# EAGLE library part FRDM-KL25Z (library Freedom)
For creating FRDM-KL25Z shields
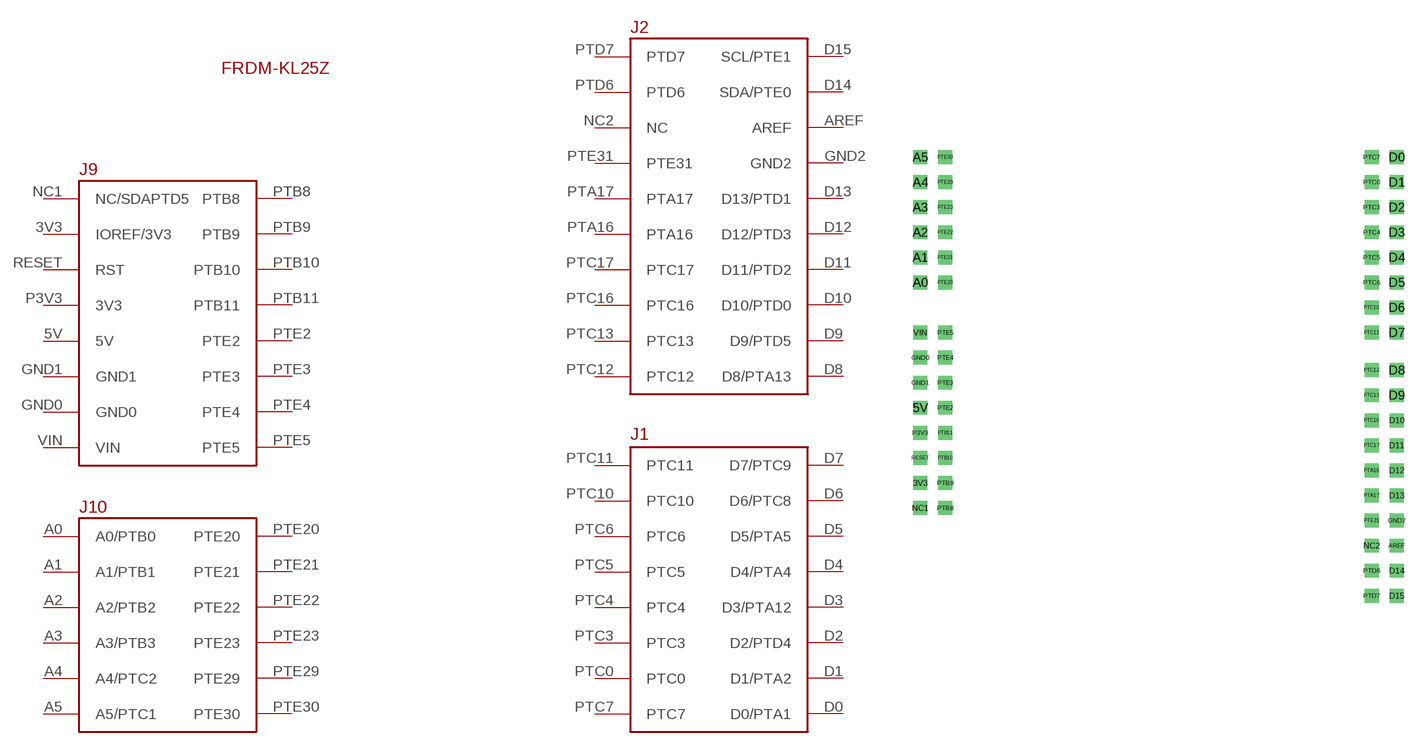
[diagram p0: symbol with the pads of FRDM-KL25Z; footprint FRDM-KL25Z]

Designator prefix FRDM

## FRDM-KL25ZARDUINO  [FRDM-KL25Z]
3V3  IOREF/3V3
5V  5V
A0  A0/PTB0
A1  A1/PTB1
A2  A2/PTB2
A3  A3/PTB3
A4  A4/PTC2
A5  A5/PTC1
AREF  AREF
D0  D0/PTA1
D1  D1/PTA2
D2  D2/PTD4
D3  D3/PTA12
D4  D4/PTA4
D5  D5/PTA5
D6  D6/PTC8
D7  D7/PTC9
D8  D8/PTA13
D9  D9/PTD5
D10  D10/PTD0
D11  D11/PTD2
D12  D12/PTD3
D13  D13/PTD1
D14  SDA/PTE0
D15  SCL/PTE1
GND0  GND0
GND1  GND1
GND2  GND2
NC1  NC/SDAPTD5
NC2  NC
P3V3  3V3
PTA16  PTA16
PTA17  PTA17
PTB8  PTB8
PTB9  PTB9
PTB10  PTB10
PTB11  PTB11
PTC0  PTC0
PTC3  PTC3
PTC4  PTC4
PTC5  PTC5
PTC6  PTC6
PTC7  PTC7
PTC10  PTC10
PTC11  PTC11
PTC12  PTC12
PTC13  PTC13
PTC16  PTC16
PTC17  PTC17
PTD6  PTD6
PTD7  PTD7
PTE2  PTE2
PTE3  PTE3
PTE4  PTE4
PTE5  PTE5
PTE20  PTE20
PTE21  PTE21
PTE22  PTE22
PTE23  PTE23
PTE29  PTE29
PTE30  PTE30
PTE31  PTE31
RESET  RST
VIN  VIN

## Footprint FRDM-KL25Z (pad centres in mm)
Use straight headers (2 6-pin and 2 8-pin) to connect to an Arduino
drill 0.9 square: 3V3 -22.86,-8.89; 5V -22.86,-1.27; A0 -22.86,11.43; A1 -22.86,13.97; A2 -22.86,16.51; A3 -22.86,19.05; A4 -22.86,21.59; A5 -22.86,24.13; AREF 25.4,-15.24; D0 25.4,24.13; D1 25.4,21.59; D2 25.4,19.05; D3 25.4,16.51; D4 25.4,13.97; D5 25.4,11.43; D6 25.4,8.89; D7 25.4,6.35; D8 25.4,2.54; D9 25.4,0; D10 25.4,-2.54; D11 25.4,-5.08; D12 25.4,-7.62; D13 25.4,-10.16; D14 25.4,-17.78; D15 25.4,-20.32; GND0 -22.86,3.81; GND1 -22.86,1.27; GND2 25.4,-12.7; NC1 -22.86,-11.43; NC2 22.86,-15.24; P3V3 -22.86,-3.81; PTA16 22.86,-7.62; PTA17 22.86,-10.16; PTB8 -20.32,-11.43; PTB9 -20.32,-8.89; PTB10 -20.32,-6.35; PTB11 -20.32,-3.81; PTC0 22.86,21.59; PTC3 22.86,19.05; PTC4 22.86,16.51; PTC5 22.86,13.97; PTC6 22.86,11.43; PTC7 22.86,24.13; PTC10 22.86,8.89; PTC11 22.86,6.35; PTC12 22.86,2.54; PTC13 22.86,0; PTC16 22.86,-2.54; PTC17 22.86,-5.08; PTD6 22.86,-17.78; PTD7 22.86,-20.32; PTE2 -20.32,-1.27; PTE3 -20.32,1.27; PTE4 -20.32,3.81; PTE5 -20.32,6.35; PTE20 -20.32,11.43; PTE21 -20.32,13.97; PTE22 -20.32,16.51; PTE23 -20.32,19.05; PTE29 -20.32,21.59; PTE30 -20.32,24.13; PTE31 22.86,-12.7; RESET -22.86,-6.35; VIN -22.86,6.35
